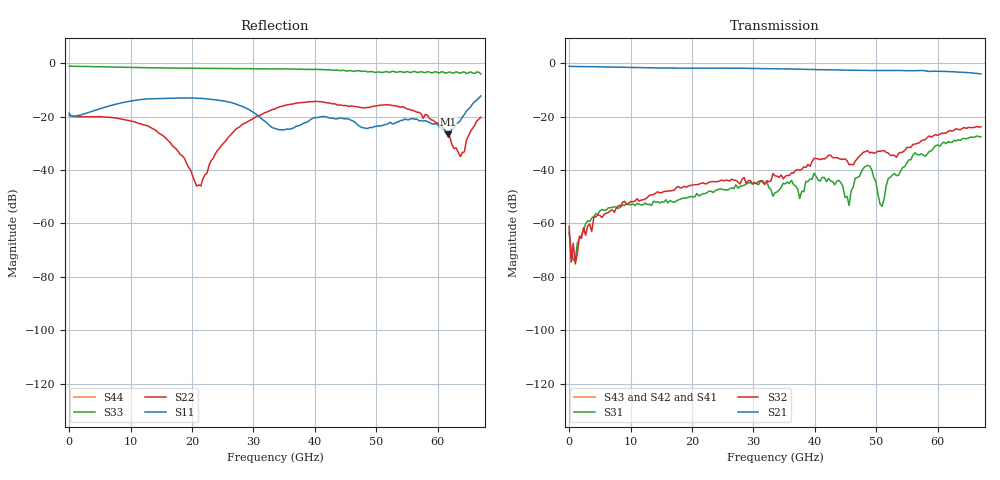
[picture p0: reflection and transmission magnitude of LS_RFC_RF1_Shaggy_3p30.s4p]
!Keysight Technologies,N5227A,US51270237,A.10.65.04
!Date: Thursday, April 28, 2022 11:36:41
!Correction: S11(Full 3 Port(1,2,3))
!S12(Full 3 Port(1,2,3))
!S13(Full 3 Port(1,2,3))
!S14(Off)
!S21(Full 3 Port(1,2,3))
!S22(Full 3 Port(1,2,3))
!S23(Full 3 Port(1,2,3))
!S24(Off)
!S31(Full 3 Port(1,2,3))
!S32(Full 3 Port(1,2,3))
!S33(Full 3 Port(1,2,3))
!S34(Off)
!S41(Off)
!S42(Off)
!S43(Off)
!S44(Off)
!S4P File: Measurements: <S11,S12,S13,S14>,
!<S21,S22,S23,S24>,
!<S31,S32,S33,S34>,
!<S41,S42,S43,S44>:
# Hz S  dB  R 50
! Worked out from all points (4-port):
!   201 points, 10 MHz to 67 GHz, reference 50 ohm
!   strongest paths, dB at 10 MHz, 16.76 GHz, 33.51 GHz, 50.25 GHz, 67 GHz:
!     S21: -1.1, -1.8, -2.1, -2.7, -4.0
!     S32: -61.0, -47.7, -42.1, -32.9, -23.8
!     S31: -63.3, -51.8, -48.5, -49.0, -27.6
!     S43: -, -, -, -, -
!     S42: -, -, -, -, -
!     S41: -, -, -, -, -
!   lowest |S11| = -26.6 dB at 61.64 GHz (marker M1), VSWR 1.10, Z = 46 + j2.07 ohm
!   |S11| at or under -10 dB: start of sweep to end of sweep
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1e7  -18.71 -0.9  -1.11 -0.2  -69.15 24.9  -200.00 45.0
     -1.09 -0.4  -19.55 -2.0  -66.35 17.8  -200.00 45.0
     -63.33 -117.3  -61.05 -129.9  -1.10 180.0  -200.00 45.0
     -200.00 45.0  -200.00 45.0  -200.00 45.0  -200.00 45.0
1.01485e9  -19.76 -16.7  -1.23 -8.5  -67.78 72.9  -200.00 45.0
           -1.21 -8.5  -19.99 -15.1  -67.99 104.5  -200.00 45.0
           -73.59 81.7  -75.17 77.7  -1.15 173.8  -200.00 45.0
           -200.00 45.0  -200.00 45.0  -200.00 45.0  -200.00 45.0
2.07769e10  -13.08 -163.5  -1.85 -162.2  -49.46 -44.0  -200.00 45.0
            -1.83 -162.0  -46.02 136.1  -45.14 -4.6  -200.00 45.0
            -48.74 -46.4  -45.47 -7.0  -1.90 52.2  -200.00 45.0
            -200.00 45.0  -200.00 45.0  -200.00 45.0  -200.00 45.0
2.848075e10  -16.43 137.8  -1.91 137.2  -46.02 -103.0  -200.00 45.0
             -1.89 137.3  -22.61 116.1  -43.57 -71.0  -200.00 45.0
             -45.73 -97.0  -42.78 -76.3  -2.02 3.9  -200.00 45.0
             -200.00 45.0  -200.00 45.0  -200.00 45.0  -200.00 45.0
4.522825e10  -20.73 -99.4  -2.61 3.5  -51.01 147.4  -200.00 45.0
             -2.59 4.0  -15.96 2.2  -36.46 152.6  -200.00 45.0
             -49.90 155.1  -36.48 150.1  -2.96 -80.8  -200.00 45.0
             -200.00 45.0  -200.00 45.0  -200.00 45.0  -200.00 45.0
6.16408e10  -26.56 151.5  -3.09 -139.8  -29.70 64.1  -200.00 45.0
            -3.11 -138.8  -26.47 -94.4  -25.52 69.6  -200.00 45.0
            -29.35 62.5  -25.54 69.0  -3.40 -179.6  -200.00 45.0
            -200.00 45.0  -200.00 45.0  -200.00 45.0  -200.00 45.0
6.7e10  -12.24 40.7  -4.00 166.0  -27.54 5.4  -200.00 45.0
        -3.98 167.1  -20.24 78.0  -23.76 19.1  -200.00 45.0
        -27.60 8.5  -23.79 15.4  -4.04 128.8  -200.00 45.0
        -200.00 45.0  -200.00 45.0  -200.00 45.0  -200.00 45.0
